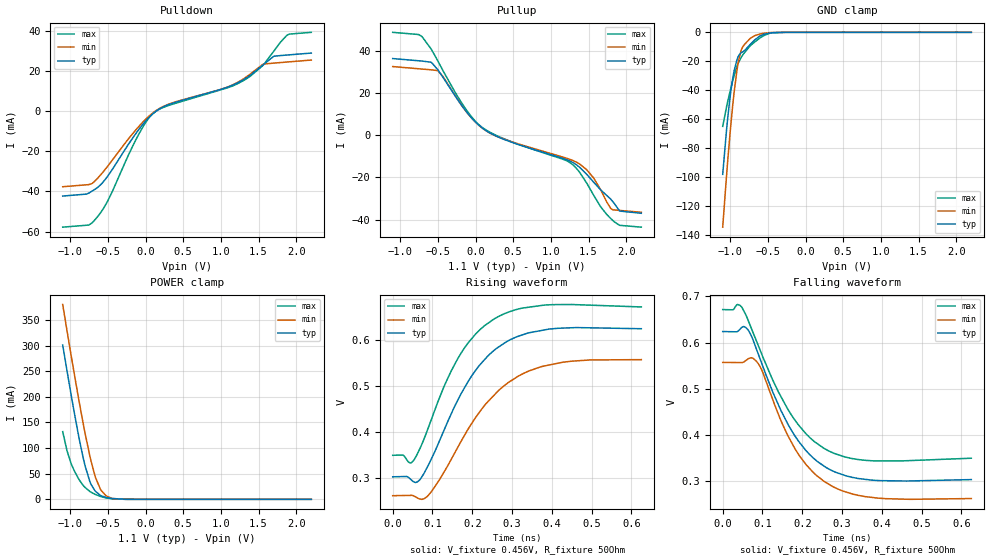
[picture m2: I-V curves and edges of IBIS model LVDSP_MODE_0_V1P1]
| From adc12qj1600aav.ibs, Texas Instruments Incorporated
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[Model]   LVDSP_MODE_0_V1P1
Model_type   3-state
Polarity   Non-Inverting
Vmeas = 0.5
Vref = 0.5
Cref = 0.2pF
Rref = 50
|   typ   min   max
C_comp   1.95pF   1.92pF   1.97pF
[Voltage Range]   1.1   1.05   1.15
[Temperature Range]   25   125   -40
[Pullup Reference]   1.1   1.05   1.15
[Pulldown Reference]   0   0   0
[Power Clamp Reference]   1.1   1.05   1.15
[GND Clamp Reference]   0   0   0
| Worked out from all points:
|   slope of the pulldown table from 0 to 0.165 V, typ, clamps not added: 29.5 ohm
|   slope of the pullup table from 0 to 0.165 V, typ, clamps not added: 35.7 ohm
|   GND clamp passes 1 mA (typ) near -0.52 V on its own axis
|   POWER clamp passes 1 mA (typ) near -0.37 V on its own axis
|   falling waveform, V_fixture 0.456V, R_fixture 50Ohm: 20-80 % time 112ps typ, 108ps min, 115ps max; typ from 0.624 V to 0.303 V
|   rising waveform, V_fixture 0.456V, R_fixture 50Ohm: 20-80 % time 123ps typ, 142ps min, 111ps max; typ from 0.303 V to 0.624 V
[Pulldown]
|   Voltage   I(typ)   I(min)   I(max)
-1.1V     -42.26mA   -37.63mA   -57.73mA
-753.5mV  -40.82mA   -36.58mA   -56.68mA
-638mV    -38.03mA   -33.47mA   -52.57mA
-506mV    -32.55mA   -27.57mA   -44.95mA
-90.2mV   -9.213mA   -7.702mA   -11.53mA
48.4mV    -3.005mA   -2.425mA   -3.261mA
137.5mV   -85.55uA   185.3uA    -111.4uA
1.226V    14.11mA    14.38mA    13.68mA
1.563V    23.08mA    23.31mA    22.89mA
1.702V    27.25mA    23.84mA    29.74mA
1.88V     27.86mA    24.38mA    37.78mA
2.2V      28.83mA    25.35mA    39.14mA
[GND Clamp]
|   Voltage   I(typ)   I(min)   I(max)
-1.1V     -97.96mA   -134.4mA   -64.87mA
-1.047V   -66.26mA   -97.58mA   -50.92mA
-997.7mV  -42.75mA   -66.86mA   -39.78mA
-951.5mV  -27.35mA   -42.75mA   -30.48mA
-911.9mV  -19.09mA   -26.62mA   -23.78mA
-885.5mV  -15.85mA   -18.64mA   -20.34mA
-852.5mV  -13.98mA   -12.11mA   -17.12mA
-806.3mV  -12.42mA   -8.08mA    -13.71mA
-730.4mV  -8.095mA   -3.993mA   -9.048mA
-605mV    -2.515mA   -1.15mA    -3.896mA
-446.6mV  -282.5uA   -128.4uA   -336uA
2.2V      0A         0A         0A
[Pullup]
|   Voltage   I(typ)   I(min)   I(max)
-1.1V     36.23mA    32.45mA    48.64mA
-710.6mV  35.05mA    31.27mA    46.59mA
-591.8mV  34.5mA     30.91mA    40.87mA
-496.1mV  30.67mA    30.33mA    34.79mA
-156.2mV  12.72mA    12.67mA    13.72mA
71.5mV    3.921mA    3.848mA    4.131mA
371.8mV   -1.898mA   -1.775mA   -1.602mA
1.25V     -12.19mA   -11.4mA    -12.89mA
1.477V    -18.58mA   -16.41mA   -22.79mA
1.824V    -31.49mA   -35.31mA   -40.38mA
1.916V    -35.89mA   -35.58mA   -42.63mA
2.2V      -36.93mA   -36.44mA   -43.49mA
[POWER Clamp]
|   Voltage   I(typ)   I(min)   I(max)
-1.1V     301.3mA    380.2mA    132.1mA
-1.044V   251.8mA    329.9mA    95.44mA
-987.8mV  203.6mA    280.6mA    69.65mA
-875.6mV  114.1mA    185.7mA    36.88mA
-799.7mV  63.62mA    126.5mA    22.8mA
-733.7mV  32.59mA    80.75mA    14.78mA
-661.1mV  15.02mA    41.11mA    9.152mA
-598.4mV  7.626mA    19.5mA     5.607mA
-522.5mV  3.63mA     6.518mA    2.676mA
-440mV    1.582mA    1.534mA    915.2uA
-275mV    131.6uA    77.51uA    29.69uA
2.2V      0A         0A         0A
[Ramp]
R_load = 50
|   typ   min   max
dV/dt_r   0.192914/1.2278e-10   0.177263/1.42205e-10   0.193251/1.11045e-10
dV/dt_f   0.192454/1.11888e-10   0.177005/1.08113e-10   0.193251/1.14439e-10
[Falling Waveform]
V_fixture = 0.456V
V_fixture_min = 0.39V
V_fixture_max = 0.514V
R_fixture = 50Ohm
C_fixture = 0F
|   Time   V(typ)   V(min)   V(max)
0s        623.8mV    557mV      671.4mV
43.03ps   628.5mV    556.6mV    680.8mV
63.23ps   627.9mV    564.2mV    649.7mV
85.76ps   583.6mV    558.4mV    601.3mV
127.2ps   489.9mV    472.9mV    516.1mV
172.6ps   410mV      384.3mV    443.2mV
208.9ps   366.3mV    336.2mV    402.8mV
254ps     332.7mV    299.8mV    371mV
390.4ps   301mV      262.9mV    343.5mV
625ps     303.1mV    262mV      349.3mV
[Rising Waveform]
V_fixture = 0.456V
V_fixture_min = 0.39V
V_fixture_max = 0.514V
R_fixture = 50Ohm
C_fixture = 0F
|   Time   V(typ)   V(min)   V(max)
0s        302.6mV    261.6mV    349.3mV
47.12ps   295.7mV    262.4mV    333.3mV
68.25ps   296.3mV    254.6mV    363.8mV
97ps      341.1mV    270.1mV    426.8mV
162.9ps   467.7mV    365.6mV    558.2mV
208ps     533.4mV    431mV      612.2mV
254ps     576.5mV    479.1mV    644.9mV
315.3ps   607.7mV    521.1mV    666.8mV
373.6ps   620.3mV    541.9mV    674.6mV
625ps     624.2mV    557.1mV    671.4mV
